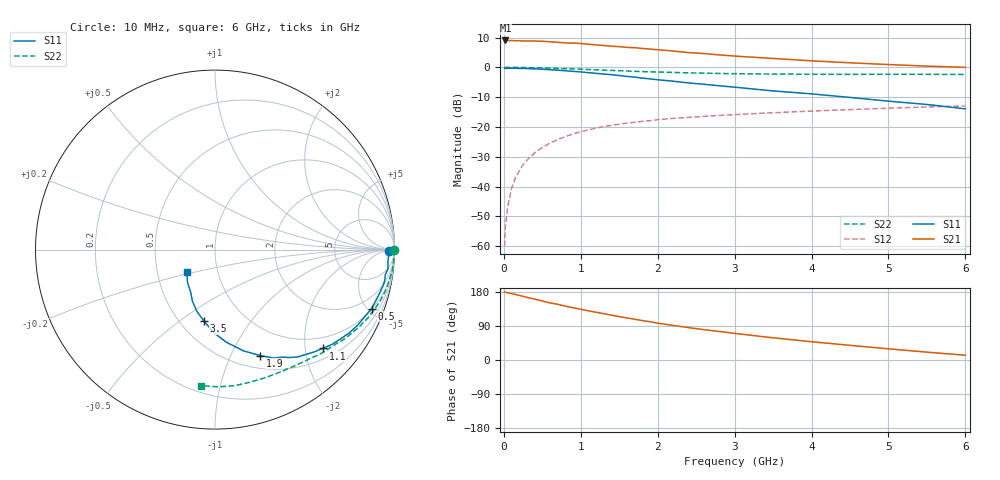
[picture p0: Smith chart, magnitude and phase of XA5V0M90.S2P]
! SIEMENS Discrete & RF Semiconductors
! BFY180
! Si NPN RF Bipolar Junction Transistor in MICRO-X
! VCE = 5 V  IC = 0.9 mA
! Common Emitter S-Parameters:  May  1997
# GHz  S  MA  R  50
!  f  S11  S21  S12  S22
! GHz  MAG  ANG  MAG  ANG  MAG  ANG  MAG  ANG
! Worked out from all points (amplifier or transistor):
!   36 points, 10 MHz to 6 GHz, reference 50 ohm
!   highest |S21| = 9.0 dB at 20 MHz (marker M1)
!   |S21| within 3 dB of that: start of sweep to 1.947 GHz
!   unconditionally stable (mu >= 1): 4.278 GHz to end of sweep
!   at 250 MHz: K = 0.07, MSG = 20.8 dB, |S12| = -32.7 dB
!   at 1.4 GHz: K = 0.47, MSG = 13.3 dB, |S12| = -19.5 dB
!   at 6 GHz: K = 1.04, MAG = 5.2 dB, |S12| = -12.9 dB
!   S11 on the Smith chart (normalised r, x): 10 MHz: 60, -10; 500 MHz: 1.05, -5.30; 1.1 GHz: 0.73, -2.38; 1.9 GHz: 0.65, -1.30; 3.5 GHz: 0.65, -0.62; 6 GHz: 0.71, -0.19
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0.01  0.9679 -0.3  2.823 179.4  0.001 86.3  0.9986 -0.1
0.02  0.9583 -0.8  2.832 178.7  0.0021 96.5  0.9999 -0.5
0.05  0.9683 -2.0  2.81 177.6  0.0046 86.1  0.9977 -1.2
0.1  0.9656 -4.0  2.827 175.4  0.0093 87.4  0.9966 -2.6
0.15  0.97 -6.3  2.803 173.0  0.0139 86.9  0.9971 -3.9
0.25  0.9612 -10.5  2.776 168.1  0.0233 83.1  0.9952 -6.5
0.3  0.9565 -12.5  2.78 165.4  0.0276 81.0  0.9908 -7.7
0.5  0.9327 -20.6  2.75 155.7  0.0454 75.3  0.98 -12.7
0.6  0.9129 -24.4  2.689 150.7  0.0536 72.5  0.9717 -15.0
0.9  0.8574 -35.6  2.566 138.0  0.0764 64.2  0.9423 -22.0
1.1  0.8148 -42.5  2.446 129.8  0.0894 59.8  0.921 -26.2
1.5  0.7303 -55.4  2.228 114.5  0.1116 51.3  0.8804 -33.9
1.7  0.688 -61.5  2.142 107.6  0.12 47.9  0.8579 -37.3
1.9  0.642 -66.9  2.027 101.0  0.1278 44.7  0.8421 -40.5
2.2  0.5869 -74.2  1.884 91.2  0.1396 40.5  0.8237 -45.2
2.6  0.5212 -82.8  1.708 80.1  0.1509 35.8  0.7996 -50.7
3  0.4657 -90.4  1.548 70.2  0.1613 31.7  0.7844 -56.0
3.5  0.4029 -98.8  1.413 58.6  0.1737 27.4  0.7723 -62.2
4  0.3594 -106.2  1.289 48.2  0.1849 23.1  0.7668 -68.6
4.5  0.3134 -113.7  1.194 38.7  0.1957 19.2  0.7642 -75.2
5.5  0.2386 -129.9  1.05 20.7  0.2167 11.3  0.765 -88.8
6  0.2015 -140.9  1.002 12.6  0.2256 7.1  0.761 -95.7
